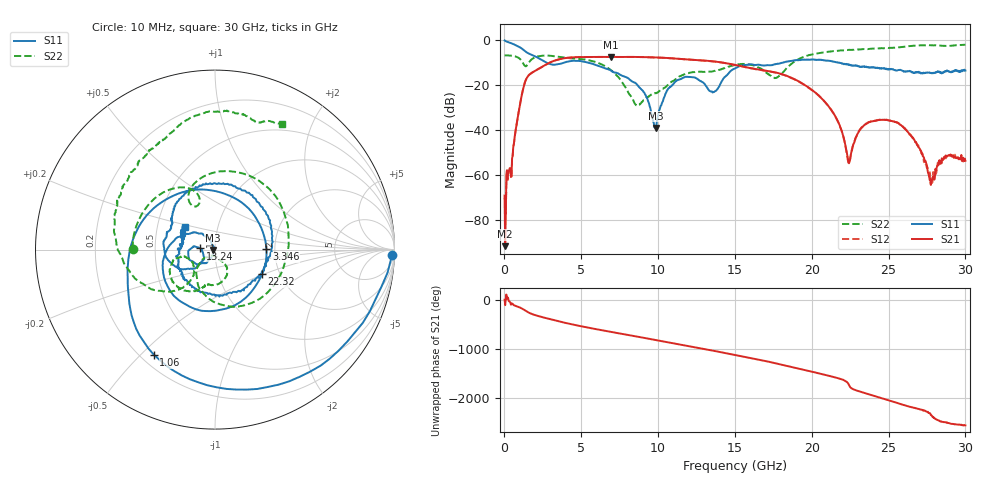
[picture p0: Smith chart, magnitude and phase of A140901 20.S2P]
!  2-Port S-parameters saved by WinCal
! VAR MeasName=S-Parameters (CALIBRATED_DATA) read from VNA (N5244A)
! VAR MeasDate=11/3/2014 9:28:26 AM
! VAR NAME=A140901 20
! VAR FILENAME=A140901 20.S2P
! VAR DATE=11/3/2014 9:28:26 AM
! VAR PHYS_PORTS=1,2
# Hz S RI R 50
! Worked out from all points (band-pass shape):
!   801 points, 10 MHz to 30 GHz, reference 50 ohm
!   highest |S21| = -7.41 dB at 6.908 GHz (marker M1); lowest = -91.6 dB at 47.49 MHz (marker M2)
!   |S21| within 3 dB of the highest: 2.823 GHz to 14.57 GHz (11.75 GHz wide, 135 % of centre)
!   lowest |S11| = -39.1 dB at 9.869 GHz (marker M3), VSWR 1.02, Z = 48.9 - j0.195 ohm
!   |S11| at or under -10 dB: 2.738 GHz to 3.853 GHz (1.115 GHz wide, 33.8 % of centre); 5.446 GHz to 18.12 GHz (12.68 GHz wide, 108 % of centre); 21.77 GHz to end of sweep
!   |S22| runs from -29.1 to -2.0 dB; largest |S21 - S12| = 0.0036
!   S11 on the Smith chart (normalised r, x): 10 MHz: 24, -56; 1.06 GHz: 0.25, -0.55; 3.346 GHz: 1.80, +0.01; 13.24 GHz: 0.85, +0.01; 22.32 GHz: 1.61, -0.48; 30 GHz: 0.69, +0.18
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1e7  0.9866 -0.0299  0.000349 2.39e-05  -0.000269 0.000164  -0.4589 0.0049
4.74875e7  0.9615 -0.1285  -8.16e-06 -2.49e-05  -0.000258 8.08e-05  -0.4586 0.0232
5.34825e8  0.3535 -0.7527  0.000388 -0.00269  0.000261 -0.00258  -0.3746 0.2452
1.05965e9  -0.3405 -0.586  -0.0442 -0.0129  -0.0443 -0.0127  -0.1392 0.3399
2.371712e9  -0.2045 0.3119  0.2381 0.0659  0.2375 0.0662  0.1126 0.4332
3.346388e9  0.2867 0.00157  0.1641 -0.3194  0.1643 -0.32  0.3884 0.1928
5.033325e9  -0.2492 -0.2308  -0.4224 0.00344  -0.422 0.00467  0.2949 -0.2369
6.9077e9  -0.2019 0.0707  0.151 0.3987  0.1509 0.3976  -0.094 -0.1976
8.594638e9  -0.0661 0.0837  0.3815 -0.1843  0.3816 -0.1836  -0.0125 -0.0339
9.869212e9  -0.011 -0.002  -0.0583 -0.4088  -0.0583 -0.4086  0.0317 -0.0588
1.001916e10  -0.0127 -0.0194  -0.1194 -0.3943  -0.1191 -0.3938  0.0331 -0.062
1.129374e10  -0.1012 -0.0829  -0.3871 0.000977  -0.3873 0.00225  0.0684 -0.1342
1.324309e10  -0.0824 0.00673  0.1406 0.3178  0.1405 0.3161  -0.0418 -0.1971
1.5005e10  -0.2149 -0.0972  0.209 -0.1901  0.2058 -0.1911  -0.1597 -0.2305
1.762912e10  -0.2403 0.1636  -0.1691 0.0914  -0.1674 0.0908  -0.1262 -0.0721
2.002832e10  0.0703 0.3668  0.0708 -0.0308  0.0709 -0.0297  -0.46 -0.1421
2.156531e10  0.3172 0.0658  -0.0152 -0.0119  -0.0149 -0.0121  -0.5608 0.1292
2.231506e10  0.2591 -0.1365  -0.00134 0.00237  -0.00138 0.00214  -0.5429 0.2645
2.34022e10  0.0295 -0.2543  -0.000375 -0.0127  -0.000354 -0.0129  -0.4749 0.4232
2.501416e10  -0.1909 -0.1123  -0.00717 0.0146  -0.00726 0.015  -0.309 0.5986
2.782572e10  -0.1736 0.0568  -0.000733 0.000305  -0.00061 0.000274  0.1119 0.7594
3e10  -0.1696 0.126  0.00171 -0.0012  0.00183 -0.0014  0.3737 0.7001
